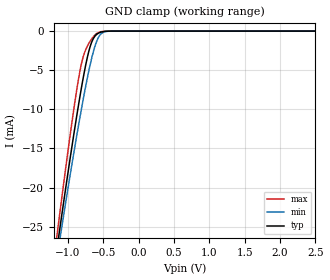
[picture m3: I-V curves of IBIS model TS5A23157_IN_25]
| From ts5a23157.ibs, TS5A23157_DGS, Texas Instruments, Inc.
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[Model]   TS5A23157_IN_25
Model_type  Input
Vinl=0.81
Vinh=1.61
| variable   typ   min   max
C_comp   2.62pF   2.11pF   3.26pF
[Temperature Range]   40   100   -40
| Ambient temperature   25   85   -40
[Voltage range]   2.5   2.3   2.7
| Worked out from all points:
|   GND clamp passes 1 mA (typ) near -0.64 V on its own axis
[GND Clamp]
| TS5A23157_IN_25
|   Voltage   I(typ)   I(min)   I(max)
-2.5V     -120.2mA   -113.2mA   -128.6mA
-1.15V    -27.47mA   -28.67mA   -25.74mA
-1.125V   -25.88mA   -27.22mA   -23.97mA
-1.085V   -23.36mA   -24.92mA   -21.17mA
-925mV    -13.66mA   -15.99mA   -10.47mA
-820mV    -7.8mA     -10.49mA   -4.628mA
-765mV    -5.061mA   -7.792mA   -2.746mA
-690mV    -2.097mA   -4.463mA   -1.35mA
-580mV    -330.5uA   -1.011mA   -236.4uA
-505mV    -70.28uA   -179.6uA   -33.48uA
-385mV    -3.196uA   -7.201uA   -526.8nA
2.5V      57.25pA    176.8pA    32.61pA
